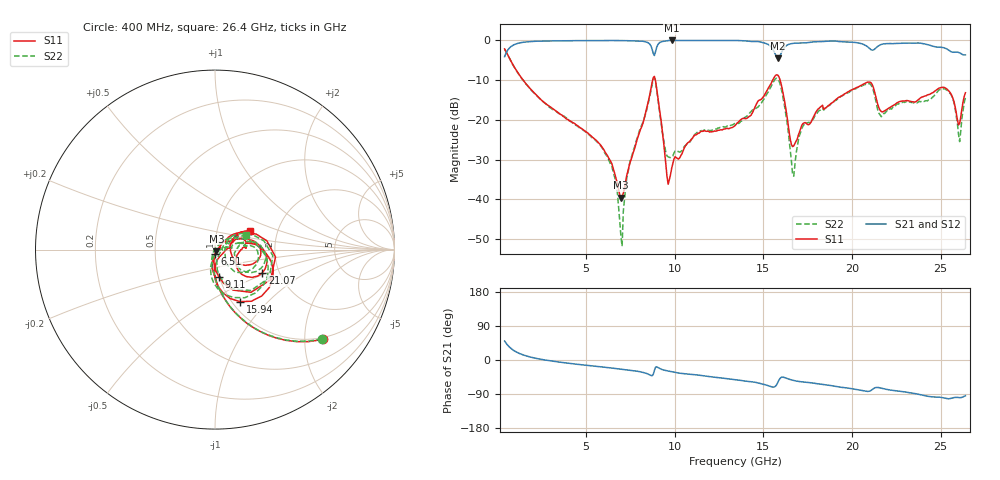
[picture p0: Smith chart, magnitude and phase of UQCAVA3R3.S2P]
!  Part Number  UQCAVA3R3 	Mounting Orientation: Horizontal
!  Description: RF capacitors
!  Application: Coupling, Bypass, Tuning, DC Block
!  Filters, Matching
# GHZ S DB R 50
! Freq  |S11|  S11 Ph  |S21|  S21 Ph  |S12|  S12 Ph  |S22|  S22 Ph
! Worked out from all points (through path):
!   401 points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, 400 MHz to 26.4 GHz, reference 50 ohm
!   highest |S21| = -0.01 dB at 9.825 GHz (marker M1); lowest = -4.5 dB at 15.8 GHz (marker M2)
!   group delay of S21, straight-line fit = 12 ps
!   lowest |S11| = -39.6 dB at 6.965 GHz (marker M3), VSWR 1.02, Z = 50.8 - j0.712 ohm
!   |S11| at or under -10 dB: 1.445 GHz to 8.754 GHz (7.309 GHz wide, 143 % of centre); 8.907 GHz to 15.53 GHz (6.619 GHz wide, 54.2 % of centre); 15.94 GHz to end of sweep
!   |S22| runs from -51.8 to -2.2 dB; largest |S21 - S12| = 0.014
!   S11 on the Smith chart (normalised r, x): 400 MHz: 0.95, -2.44; 6.51 GHz: 1.00, -0.05; 9.11 GHz: 1.00, -0.31; 15.94 GHz: 1.09, -0.70; 21.07 GHz: 1.63, -0.46; 26.4 GHz: 1.44, +0.32
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0.4  -2.14 -39.8  -4.10 50.0  -4.15 50.0  -2.19 -40.0
1.505  -10.36 -77.1  -0.44 12.5  -0.48 12.5  -10.42 -77.2
4.755  -22.22 -100.8  -0.05 -12.7  -0.07 -12.4  -22.31 -103.4
6.51  -31.95 -91.3  -0.02 -21.7  -0.02 -21.4  -32.81 -117.5
6.965  -39.60 -42.1  -0.05 -24.1  -0.03 -23.9  -49.45 -158.5
7.42  -31.71 28.4  -0.07 -26.7  -0.06 -26.4  -31.83 52.6
8.72  -10.66 9.6  -2.15 -41.5  -2.12 -41.1  -11.15 10.1
9.11  -16.39 -82.2  -0.70 -21.2  -0.66 -20.9  -16.97 -81.1
9.565  -34.35 -67.8  -0.09 -28.5  -0.05 -28.2  -29.11 -52.6
9.825  -32.23 7.8  -0.01 -30.9  -0.01 -30.6  -29.20 -18.1
11.19  -23.82 43.5  -0.01 -39.1  -0.01 -39.1  -23.49 29.9
13.4  -21.47 32.3  -0.01 -51.9  -0.01 -52.0  -20.91 36.6
15.22  -12.49 5.3  -0.90 -66.8  -0.86 -67.1  -13.37 11.5
15.805  -8.71 -44.8  -4.51 -60.2  -4.47 -60.5  -9.63 -47.1
15.935  -9.85 -64.3  -3.92 -48.8  -3.89 -49.0  -10.86 -68.9
16.65  -26.74 -44.6  -0.76 -53.4  -0.72 -53.6  -33.73 -57.3
17.755  -19.93 27.4  -0.39 -60.5  -0.34 -60.8  -20.12 13.1
21.07  -10.65 -26.3  -2.31 -80.4  -2.26 -81.0  -11.20 -22.7
22.11  -16.94 -1.8  -0.79 -78.9  -0.76 -79.5  -17.38 8.1
25.23  -11.88 -9.2  -1.92 -100.7  -1.88 -101.5  -12.14 -18.7
26.075  -20.96 14.9  -3.13 -99.3  -3.10 -100.1  -25.48 -2.8
26.4  -13.18 28.6  -3.66 -94.3  -3.64 -95.1  -14.42 24.9
